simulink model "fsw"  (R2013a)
settings: Solver=ode45  StartTime=0.0  StopTime=200  RelTol=1e-3
libraries: simulink x5, realtime_pacer_lib x1

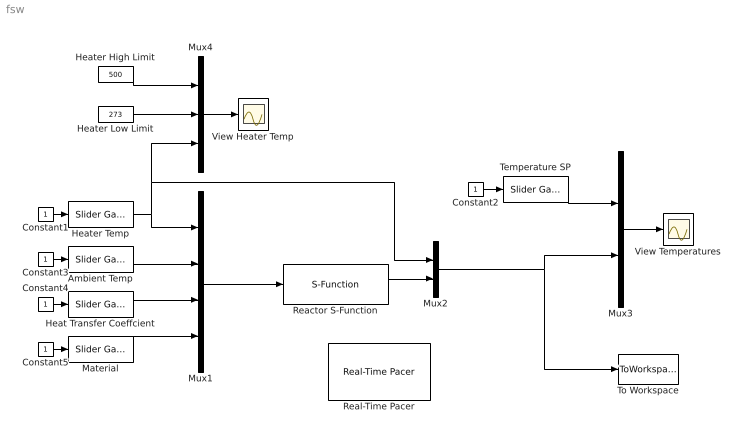
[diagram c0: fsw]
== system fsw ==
  Ambient Temp : simulink/Math Operations/Slider Gain  low=273  gain=300  high=320
  Constant{1..5} (5 alike) : Constant
  Heat Transfer Coeffcient : simulink/Math Operations/Slider Gain  low=0  gain=100  high=1000
  Heater High Limit : Constant  Value=500
  Heater Low Limit : Constant  Value=273
  Heater Temp : simulink/Math Operations/Slider Gain  low=273  gain=350  high=500
  Material : simulink/Math Operations/Slider Gain  low=0  gain=0  high=1
  Mux1 : Mux
  Mux2 : Mux  Inputs=2
  Mux3 : Mux  Inputs=2
  Mux4 : Mux  Inputs=3
  Reactor S-Function : S-Function  FunctionName=rod  EnableBusSupport=off
  Real-Time Pacer : realtime_pacer_lib/Real-Time Pacer  simTimePerRealTime=3
  Temperature SP : simulink/Math Operations/Slider Gain  low=280  gain=380  high=400
  To Workspace : ToWorkspace  VariableName=results  SampleTime=0.5  SaveFormat=Timeseries
  View Heater Temp : Scope
  View Temperatures : Scope
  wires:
  Mux1/1 -> Reactor S-Function/1
  Constant2/1 -> Temperature SP/1
  Temperature SP/1 -> Mux3/1
  Mux3/1 -> View Temperatures/1
  Heater Temp/1 -> Mux2/1, Mux4/3, Mux1/1
  Heater High Limit/1 -> Mux4/1
  Heater Low Limit/1 -> Mux4/2
  Mux4/1 -> View Heater Temp/1
  Constant1/1 -> Heater Temp/1
  Constant3/1 -> Ambient Temp/1
  Ambient Temp/1 -> Mux1/2
  Constant4/1 -> Heat Transfer Coeffcient/1
  Heat Transfer Coeffcient/1 -> Mux1/3
  Constant5/1 -> Material/1
  Material/1 -> Mux1/4
  Reactor S-Function/1 -> Mux2/2
  Mux2/1 -> To Workspace/1, Mux3/2
